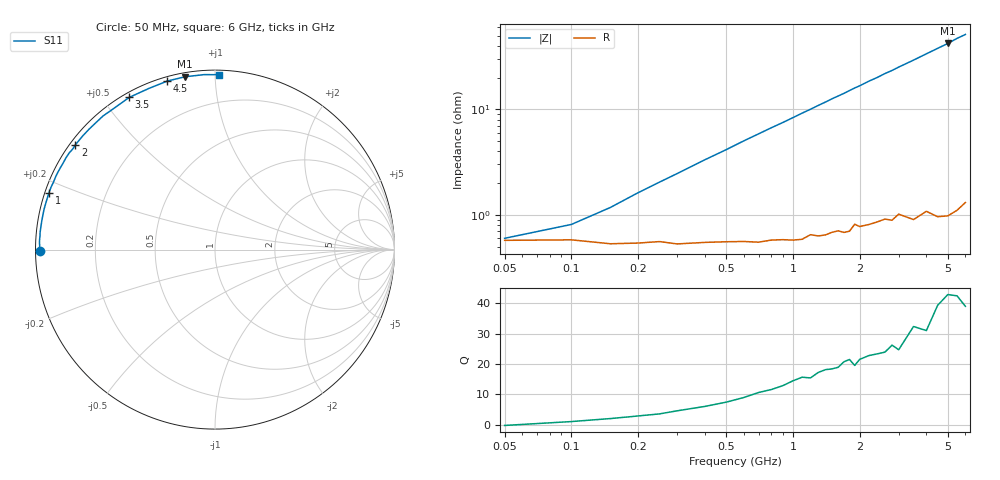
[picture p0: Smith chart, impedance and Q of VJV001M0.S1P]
! Infineon Technologies  Discrete & RF Semiconductors
! BB 914
! Si Tuning Diode in SOT23
! VR =
! S-Parameters:  July  1999
# GHz  S  MA  R  50
!  f  S11
! GHz  MAG  ANG
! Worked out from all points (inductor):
!   34 points, 50 MHz to 6 GHz, reference 50 ohm
!   read as one part to ground: L = 1.27 nH near 250 MHz
!   highest Q = 42.5 at 5 GHz (marker M1), where L = 1.34 nH
!   S11 on the Smith chart (normalised r, x): 50 MHz: 0.01, -0.00; 1 GHz: 0.01, +0.17; 2 GHz: 0.02, +0.33; 3.5 GHz: 0.02, +0.58; 4.5 GHz: 0.02, +0.76; 6 GHz: 0.03, +1.02
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0.05  0.9773 -179.6
0.1  0.9771 178.7
0.15  0.9789 177.6
0.2  0.9786 176.5
0.3  0.979 174.5
0.5  0.9781 170.6
0.7  0.9785 166.7
0.8  0.9776 164.8
1  0.9778 161.1
1.3  0.9761 155.5
1.4  0.9758 153.7
1.5  0.9746 151.8
1.6  0.974 150.1
1.7  0.9751 148.4
1.8  0.9746 146.5
1.9  0.9708 144.7
2  0.9725 143.1
2.2  0.9719 139.5
2.4  0.9709 136.4
2.6  0.9698 132.9
2.8  0.9712 130.0
3  0.9681 126.7
3.5  0.9734 119.4
4  0.9706 112.3
4.5  0.9759 105.8
5  0.9773 99.9
5.5  0.9768 93.6
6  0.9747 88.7
